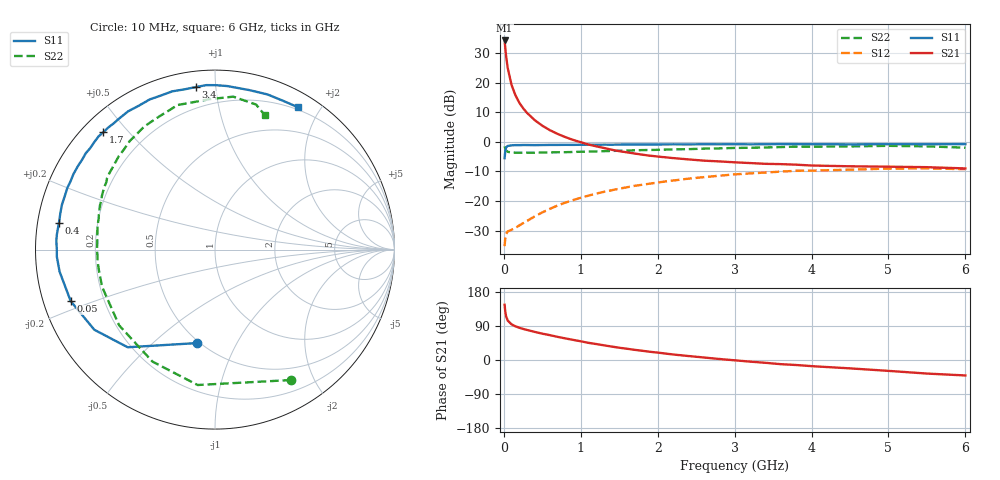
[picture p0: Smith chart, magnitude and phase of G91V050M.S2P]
! SIEMENS Small Signal Semiconductors
! BFG235
! Si NPN RF Bipolar Junction Transistor in SOT223
! VCE = 1 V  IC = 50 mA
! Common Emitter S-Parameters:  July  1994
# GHz  S  MA  R  50
!  f  S11  S21  S12  S22
! GHz  MAG  ANG  MAG  ANG  MAG  ANG  MAG  ANG
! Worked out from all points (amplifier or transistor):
!   40 points, 10 MHz to 6 GHz, reference 50 ohm
!   highest |S21| = 34.3 dB at 10 MHz (marker M1)
!   |S21| within 3 dB of that: start of sweep to 20.57 MHz
!   unconditionally stable (mu >= 1): 472.1 MHz to 1.692 GHz; 1.724 GHz to 1.922 GHz
!   at 200 MHz: K = 0.69, MSG = 20.8 dB, |S12| = -28.2 dB
!   at 1.5 GHz: K = 1.02, MAG = 5.5 dB, |S12| = -15.8 dB
!   at 6 GHz: K = 0.96, MSG = 0.1 dB, |S12| = -9.2 dB
!   S11 on the Smith chart (normalised r, x): 10 MHz: 0.48, -0.70; 50 MHz: 0.08, -0.17; 400 MHz: 0.06, +0.08; 1.7 GHz: 0.06, +0.43; 3.4 GHz: 0.08, +0.88; 6 GHz: 0.17, +1.73
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0.01  0.5308 -101.1  51.75 145.7  0.0173 57.1  0.8416 -59.7
0.02  0.7299 -131.8  37.25 125.9  0.0249 40.1  0.7606 -97.3
0.03  0.8071 -146.4  27.79 114.9  0.028 32.3  0.7146 -119.2
0.05  0.8535 -160.3  17.82 104.3  0.0307 25.2  0.6807 -141.7
0.1  0.8745 -171.9  9.221 94.2  0.0327 25.8  0.6623 -161.7
0.15  0.882 -177.4  6.171 88.9  0.0352 31.2  0.6571 -169.7
0.2  0.8815 179.6  4.613 85.2  0.0387 35.5  0.6573 -174.1
0.25  0.8855 176.8  3.716 82.0  0.0423 39.3  0.6558 -177.2
0.3  0.885 174.5  3.105 79.4  0.0461 43.2  0.6579 -179.8
0.4  0.8822 170.3  2.341 74.2  0.055 47.5  0.6568 176.4
0.5  0.8852 166.7  1.876 69.5  0.0643 50.5  0.6601 173.4
0.6  0.8887 163.7  1.573 65.5  0.074 51.9  0.664 170.5
0.7  0.8887 159.9  1.363 61.0  0.0842 53.0  0.6685 167.9
0.9  0.8903 154.7  1.081 53.1  0.1037 52.1  0.6757 163.3
1.1  0.8944 148.2  0.903 45.3  0.1236 50.4  0.6872 158.7
1.7  0.9025 133.6  0.636 26.8  0.1808 41.8  0.7218 146.4
2.2  0.9098 122.2  0.533 14.6  0.2226 33.0  0.7466 136.0
3.2  0.9089 100.9  0.439 -4.3  0.2934 13.9  0.7959 116.5
3.4  0.9117 96.8  0.426 -7.4  0.3037 9.9  0.8052 112.3
4.5  0.909 77.8  0.387 -22.1  0.3393 -10.2  0.839 91.9
5.5  0.9118 65.1  0.374 -35.8  0.3564 -27.8  0.84 74.2
6  0.9182 59.6  0.356 -40.8  0.3461 -34.4  0.7983 69.6
